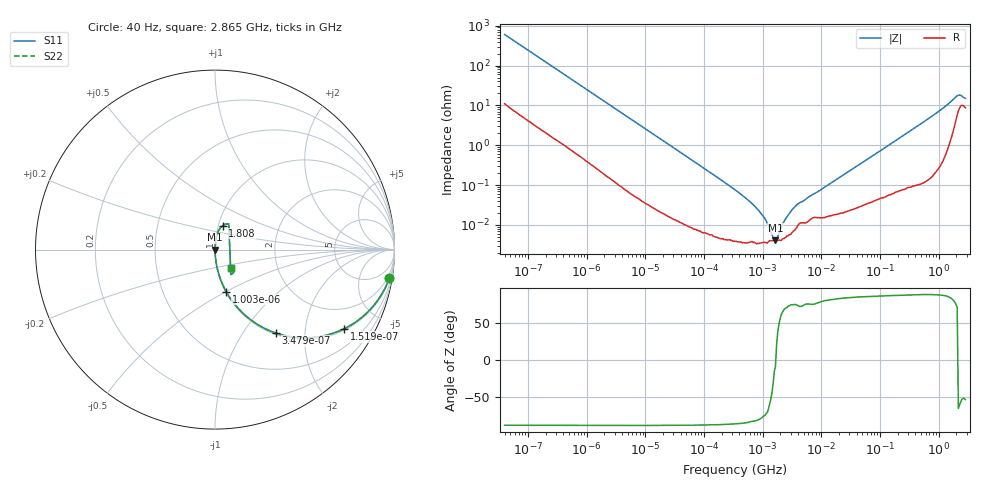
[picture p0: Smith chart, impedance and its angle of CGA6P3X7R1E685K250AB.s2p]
! S-parameter Generated by TDK Corporation
! Copyright(C) 2015 TDK Corporation.
! All Rights Reserved.
! TDK P/N: CGA6P3X7R1E685K250AB (Multilayer Ceramic Chip Capacitors)
! Property: C=6.8uF
! Size(LxWxT): 3.2x2.5x2.5mm, 0.126x0.098x0.098inches
! Model Type: s2p (Touchstone File Format Version 1.0)
! Frequency: DC=Yes Start=0.00004MHz Stop=3000MHz 396points Log-sweep
! Note: This model was converted from impedance.
! Model Generated on Jun. 23, 2015
! Hash(MD5):
! Port Assignments:
!  1 ---| |--- 2
! Applicable Conditions:
!  Temperature = 25 degC
!  DC Bias Voltage = 0 V
!  Small Signal Operation
! Terms and conditions regarding TDK Simulation Models
! (1)This simulation model is being provided solely for informational purposes. Please refer to the specifications of the products in terms of detailed characteristics of such products.
! (2)In no event shall TDK Corporation of any of its subsidiaries be liable for any loss or damage arising, directly or indirectly,
!  From any information contained in this simulation model, including, but not limited to loss or damages arising from any inaccuracies, omissions or errors in connection with such information.
! (3)Any and all copyrights on this simulation model are owned by TDK Corporation.
!  Duplication or redistribution of this simulation model without prior written permission from TDK Corporation is prohibited.
! (4)This simulation model is subject to any modification or change without any prior notice.
! (5)Neither TDK Corporation nor any of its subsidiaries shall make any warranty, express or implied,
!  Including but not limited to the correctness, implied warranties of merchantability and fitness for a particular purpose with respect to this simulation models.
! (6)The use of this simulation model shall be deemed to have consented to the terms and conditions hereof.
# MHz S MA R 50
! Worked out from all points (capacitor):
!   394 points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, 40 Hz to 2.865 GHz, reference 50 ohm
!   read as one part in series: C = 6.59 uF near 41.88 Hz
!   lowest |Z| = 4.12 mohm at 1.656 MHz (marker M1)
!   series resonance near 1.68 MHz, so ESL is about 1.4 nH
!   S11 on the Smith chart (normalised r, x): 40 Hz: 1, -12; 151.9 Hz: 1.05, -3.23; 347.9 Hz: 1.02, -1.42; 1.003 kHz: 1.01, -0.50; 1.808 GHz: 1.05, +0.29; 2.865 GHz: 1.18, -0.24
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4e-05  0.9835 -9.4  0.1636 79.5  0.1636 79.5  0.9835 -9.4
8.353326e-05  0.941 -18.8  0.3227 70.2  0.3227 70.2  0.941 -18.8
0.0001519485  0.8438 -31.5  0.5228 57.5  0.5228 57.5  0.8438 -31.5
0.0003479132  0.5752 -53.9  0.8084 35.1  0.8084 35.1  0.5752 -53.9
0.000834128  0.2864 -72.4  0.9535 16.6  0.9535 16.6  0.2864 -72.4
0.001002727  0.2422 -75.1  0.9664 14.0  0.9664 14.0  0.2422 -75.1
0.003168613  0.08061 -84.6  0.9956 4.6  0.9956 4.6  0.08061 -84.6
0.01739424  0.01504 -88.3  0.9997 0.9  0.9997 0.9  0.01504 -88.3
0.3464102  0.0007426 -87.0  1 0.0  1 0.0  0.0007426 -87.0
0.7234193  0.0003041 -83.1  1 0.0  1 0.0  0.0003041 -83.1
0.9983948  0.0001742 -78.0  1 0.0  1 0.0  0.0001742 -78.0
1.256723  9.824e-05 -67.1  1 0.0  1 0.0  9.824e-05 -67.1
1.656397  4.116e-05 -9.3  1 0.0  1 0.0  4.116e-05 -9.3
2.183178  0.0001036 64.3  1 -0.0  1 -0.0  0.0001036 64.3
3.622024  0.0002976 74.8  0.9999 -0.0  0.9999 -0.0  0.0002976 74.8
7.22376  0.0005861 75.0  0.9998 -0.0  0.9998 -0.0  0.0005861 75.0
143.8628  0.0102 86.2  0.9994 -0.6  0.9994 -0.6  0.0102 86.2
687.8953  0.04754 85.6  0.9975 -2.7  0.9975 -2.7  0.04754 85.6
1808.253  0.14 72.1  0.9663 -7.9  0.9663 -7.9  0.14 72.1
2075.972  0.1631 62.0  0.9347 -8.9  0.9347 -8.9  0.1631 62.0
2173.747  0.1649 -57.5  0.922 8.7  0.922 8.7  0.1649 -57.5
2865.06  0.137 -47.9  0.9138 6.4  0.9138 6.4  0.137 -47.9
